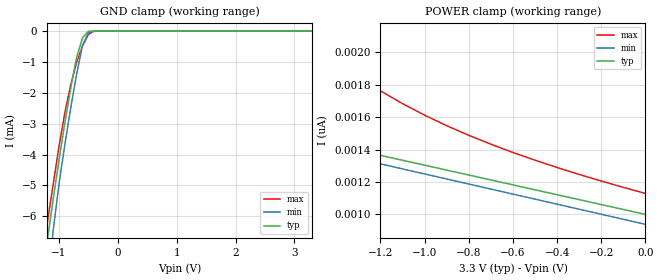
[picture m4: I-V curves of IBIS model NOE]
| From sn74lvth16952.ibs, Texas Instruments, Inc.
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|   LVTH16952 N_OE
[Model]   NOE
| Signals
Model_type  Input
Polarity   Inverting
Vinl = 0.8V
Vinh = 2.0V
| variable   typ   min   max
C_comp   4p   NA   NA
[Temperature Range]   50   100   0
[Voltage range]   3.3   3   3.6
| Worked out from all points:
|   GND clamp passes 1 mA (typ) near -0.71 V on its own axis
|Process range|   weak   strong
[GND Clamp]
|   50C:3.3V:   100C:3V:weak   0C:3.6V:strong
|   Voltage   I(typ)   I(min)   I(max)
-3.3V     -82.56mA   -87.25mA   -78mA
-1.3V     -8.397mA   -11.24mA   -7.565mA
-1.2V     -6.802mA   -8.589mA   -6.234mA
-1.1V     -5.466mA   -6.489mA   -4.985mA
-1V       -4.185mA   -4.956mA   -3.74mA
-900mV    -2.972mA   -3.679mA   -2.645mA
-800mV    -1.847mA   -2.485mA   -1.736mA
-700mV    -850.9uA   -1.396mA   -1.012mA
-600mV    -217.5uA   -464.6uA   -483.6uA
-500mV    -3.493uA   -47.69uA   -105.5uA
-400mV    -97.59nA   -2.379uA   -778.4nA
3.3V      1.001nA    1.033nA    1.023nA
[POWER Clamp]
|   50C:3.3V:   100C:3V:weak   0C:3.6V:strong
|   Voltage   I(typ)   I(min)   I(max)
-3.3V     2.004nA    1.964nA    13nA
-1.6V     1.486nA    1.436nA    2.185nA
-1.5V     1.456nA    1.405nA    2.059nA
-1.4V     1.426nA    1.374nA    1.948nA
-1.3V     1.395nA    1.343nA    1.85nA
-1.2V     1.365nA    1.312nA    1.762nA
-1.1V     1.334nA    1.281nA    1.684nA
-900mV    1.274nA    1.219nA    1.548nA
-700mV    1.213nA    1.157nA    1.433nA
-500mV    1.152nA    1.095nA    1.335nA
-300mV    1.092nA    1.033nA    1.247nA
0V        1.001nA    939.4pA    1.13nA
